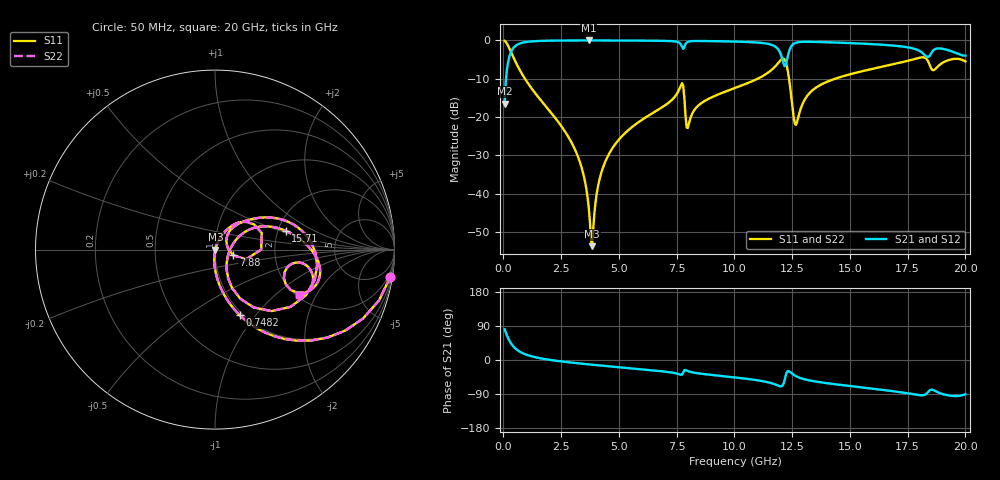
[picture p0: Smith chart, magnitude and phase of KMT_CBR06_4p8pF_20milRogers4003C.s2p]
! Data measured by Modelithics Inc. support@modelithics.com 813-866-6335
! KEMET CBR0603 4.8pF, Pad Width= 0.851mm, Pad Length= 0.64mm, Pad Gap= 0.62mm, 20mil Rogers 4003C substrate Data, January 2022
# hz S ma R 50
! 2 Port Network Data from SP1.SP block
! freq  magS11  angS11  magS21  angS21  magS12  angS12  magS22  angS22
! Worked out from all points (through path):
!   401 points, 50 MHz to 20 GHz, reference 50 ohm
!   highest |S21| = -0.02 dB at 3.691 GHz (marker M1); lowest = -16.5 dB at 50 MHz (marker M2)
!   group delay of S21, straight-line fit = 15.8 ps
!   lowest |S11| = -53.6 dB at 3.841 GHz (marker M3), VSWR 1.00, Z = 50.2 + j0.0281 ohm
!   |S11| at or under -10 dB: 930.2 MHz to 11 GHz (10.07 GHz wide, 169 % of centre); 12.36 GHz to 14.36 GHz (1.995 GHz wide, 14.9 % of centre)
!   |S22| runs from -53.6 to -0.1 dB; largest |S21 - S12| = 0
!   S11 on the Smith chart (normalised r, x): 50 MHz: 1, -13; 748.2 MHz: 0.97, -0.83; 7.88 GHz: 1.22, -0.08; 15.71 GHz: 2.21, +0.55; 20 GHz: 2.06, -1.45
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5e7  0.9886 -8.8  0.1503 81.2  0.1503 81.2  0.9886 -8.8
2.99375e8  0.7372 -43.4  0.6749 46.5  0.6749 46.5  0.7372 -43.4
7.4825e8  0.3896 -69.4  0.92 20.5  0.92 20.5  0.3896 -69.4
2.74325e9  0.05956 -93.9  0.9965 -5.5  0.9965 -5.5  0.05956 -93.9
3.391625e9  0.02161 -94.9  0.9978 -9.8  0.9978 -9.8  0.02161 -94.9
3.690875e9  0.006715 -85.1  0.9979 -11.6  0.9979 -11.6  0.006715 -85.1
3.8405e9  0.002078 7.7  0.9979 -12.5  0.9979 -12.5  0.002078 7.7
4.13975e9  0.01456 67.8  0.9977 -14.2  0.9977 -14.2  0.01456 67.8
4.588625e9  0.03393 69.6  0.9971 -16.8  0.9971 -16.8  0.03393 69.6
6.73325e9  0.1268 59.3  0.988 -29.0  0.988 -29.0  0.1268 59.3
7.680875e9  0.2595 32.5  0.8866 -39.0  0.8866 -39.0  0.2595 32.5
7.880375e9  0.1067 -17.5  0.8941 -26.3  0.8941 -26.3  0.1067 -17.5
8.03e9  0.08242 39.4  0.9681 -30.3  0.9681 -30.3  0.08242 39.4
1.0025e10  0.2396 42.6  0.9648 -46.0  0.9648 -46.0  0.2396 42.6
1.172075e10  0.4433 19.9  0.8464 -63.5  0.8464 -63.5  0.4433 19.9
1.206988e10  0.5753 -8.6  0.5772 -68.3  0.5772 -68.3  0.5753 -8.6
1.226938e10  0.4651 -47.4  0.5435 -32.0  0.5435 -32.0  0.4651 -47.4
1.266838e10  0.07957 -9.7  0.932 -42.8  0.932 -42.8  0.07957 -9.7
1.336662e10  0.222 30.3  0.9575 -55.3  0.9575 -55.3  0.222 30.3
1.571075e10  0.4081 14.8  0.9022 -73.7  0.9022 -73.7  0.4081 14.8
1.670825e10  0.4765 7.1  0.8641 -81.1  0.8641 -81.1  0.4765 7.1
2e10  0.531 -28.5  0.6331 -90.5  0.6331 -90.5  0.531 -28.5
